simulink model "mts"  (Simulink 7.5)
settings: Solver=FixedStepDiscrete  StartTime=1  StopTime=num(end)  FixedStep=1  RelTol=1e-3
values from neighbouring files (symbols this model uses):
  high = data{2}    [priceTxt.m]
  low = data{3}    [priceTxt.m]
  spread = data{5}    [priceTxt.m]
undefined symbols (not defined in the file or in its folder): sl, tp
libraries: dspsrcs4 x4, dspsigops x1

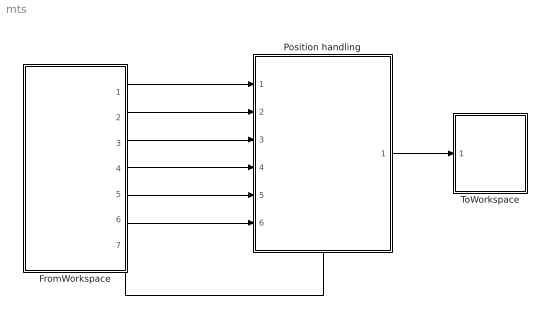
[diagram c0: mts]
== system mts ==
  FromWorkspace : Subsystem
  Position handling : Stateflow chart  TreatAsAtomicUnit=on
  ToWorkspace : Subsystem
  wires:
  FromWorkspace/1(price) -> Position handling/1(Input)
  FromWorkspace/2(spread) -> Position handling/2(spread)
  FromWorkspace/3(high) -> Position handling/3(high)
  FromWorkspace/4(low) -> Position handling/4(low)
  FromWorkspace/5(tp) -> Position handling/5(tp)
  FromWorkspace/6(sl) -> Position handling/6(sl)
  FromWorkspace/7(Buy/Sell) -> Position handling/Trigger
  Position handling/1(Output) -> ToWorkspace/1(In1)

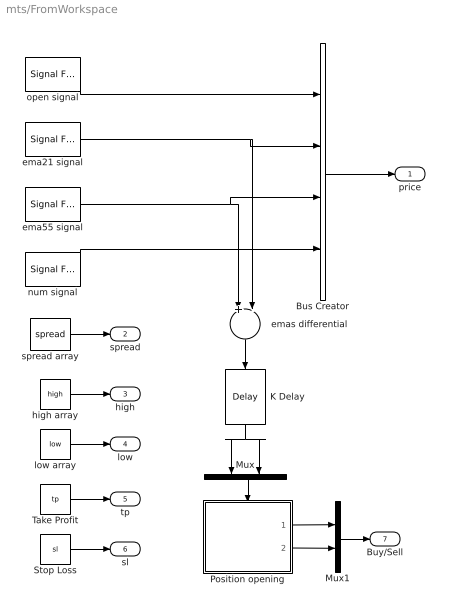
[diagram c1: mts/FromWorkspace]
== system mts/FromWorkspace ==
  Bus Creator : BusCreator  UseBusObject=on
  K Delay : dspsigops/Delay  dly_unit=Samples  delay=K  ic_detail=off  dif_ic_for_ch=off  dif_ic_for_dly=off  ic=0  reset_popup=None
  Mux : Mux  Inputs=2
  Mux1 : Mux  Inputs=2
  Position opening : Stateflow chart  TreatAsAtomicUnit=on
  Stop Loss : Constant  Value=sl  OutDataType=fixdt(1, 16)  OutScaling=2^0
  Take Profit : Constant  Value=tp  OutDataType=fixdt(1, 16)  OutScaling=2^0
  ema21 signal : dspsrcs4/Signal From Workspace  SystemSampleTime=-1  X=ema21  Ts=1  nsamps=1  OutputAfterFinalValue=Holding final value  ignoreOrWarnInputAndFrameLengths=off
  ema55 signal : dspsrcs4/Signal From Workspace  SystemSampleTime=-1  X=ema55  Ts=1  nsamps=1  OutputAfterFinalValue=Holding final value  ignoreOrWarnInputAndFrameLengths=off
  emas differential : Sum  Inputs=+-  OutDataType=fixdt(1, 16)  OutScaling=2^-10
  high array : Constant  Value=high  OutDataType=fixdt(1, 16)  OutScaling=2^0
  low array : Constant  Value=low  OutDataType=fixdt(1, 16)  OutScaling=2^0
  num signal : dspsrcs4/Signal From Workspace  SystemSampleTime=-1  X=num  Ts=1  nsamps=1  OutputAfterFinalValue=Holding final value  ignoreOrWarnInputAndFrameLengths=off
  open signal : dspsrcs4/Signal From Workspace  SystemSampleTime=-1  X=open  Ts=1  nsamps=1  OutputAfterFinalValue=Setting to zero  ignoreOrWarnInputAndFrameLengths=off
  spread array : Constant  Value=spread  OutDataType=fixdt(1, 16)  OutScaling=2^0
  price : Outport  OutDataType=fixdt(1, 16)  OutScaling=2^0
  spread : Outport  Port=2  OutDataType=fixdt(1, 16)  OutScaling=2^0
  high : Outport  Port=3  OutDataType=fixdt(1, 16)  OutScaling=2^0
  low : Outport  Port=4  OutDataType=fixdt(1, 16)  OutScaling=2^0
  tp : Outport  Port=5  OutDataType=fixdt(1, 16)  OutScaling=2^0
  sl : Outport  Port=6  OutDataType=fixdt(1, 16)  OutScaling=2^0
  Buy/Sell : Outport  Port=7  OutDataType=fixdt(1, 16)  OutScaling=2^0
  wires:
  open signal/1 -> Bus Creator/1
  ema21 signal/1 -> Bus Creator/2, emas differential/2
  ema55 signal/1 -> Bus Creator/3, emas differential/1
  num signal/1 -> Bus Creator/4
  spread array/1 -> spread/1
  high array/1 -> high/1
  low array/1 -> low/1
  Take Profit/1 -> tp/1
  Stop Loss/1 -> sl/1
  Bus Creator/1 -> price/1
  emas differential/1 -> K Delay/1
  K Delay/1 -> Mux/2, Mux/1
  Mux/1 -> Position opening/Trigger
  Position opening/1(OpenBuy) -> Mux1/1
  Position opening/2(OpenSell) -> Mux1/2
  Mux1/1 -> Buy/Sell/1

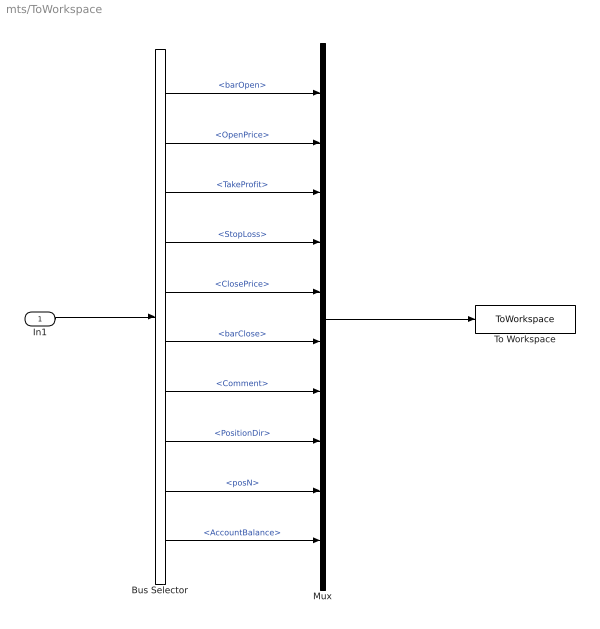
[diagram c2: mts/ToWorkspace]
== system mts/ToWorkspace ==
  In1 : Inport
  Bus Selector : BusSelector  OutputSignals=barOpen,OpenPrice,TakeProfit,StopLoss,ClosePrice,barClose,Comment,PositionDir,posN,AccountBalance
  Mux : Mux  Inputs=10
  To Workspace : ToWorkspace  VariableName=AccountBalance  SampleTime=-1  SaveFormat=Array
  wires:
  In1/1 -> Bus Selector/1
  Mux/1 -> To Workspace/1
  Bus Selector/1 -> Mux/1  "<barOpen>"
  Bus Selector/2 -> Mux/2  "<OpenPrice>"
  Bus Selector/3 -> Mux/3  "<TakeProfit>"
  Bus Selector/4 -> Mux/4  "<StopLoss>"
  Bus Selector/5 -> Mux/5  "<ClosePrice>"
  Bus Selector/6 -> Mux/6  "<barClose>"
  Bus Selector/7 -> Mux/7  "<Comment>"
  Bus Selector/8 -> Mux/8  "<PositionDir>"
  Bus Selector/9 -> Mux/9  "<posN>"
  Bus Selector/10 -> Mux/10  "<AccountBalance>"

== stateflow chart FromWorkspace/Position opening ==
  (default) -> (junction 3)
  (junction 3) -> (junction 4) : Buy{OpenBuy;}
  (junction 3) -> (junction 5) : {OpenSell;}

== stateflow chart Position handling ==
  state Position handling [group]
  (junction 16) -> (junction 17) : {Output.AccountBalance = 100000;}%3
  (default) -> (junction 16) : [Input.num>=56 && Input.num>Output.barClose] {Output.barOpen=Input.num; i = Input.num-1; Output.posN++;}%1
  (junction 16) -> (junction 17) : [Output.posN!=1]%2
  (junction 17) -> (junction 18) : OpenSell {Output.PositionDir=-1; Output.OpenPrice=Input.open; Output.StopLoss=Output.OpenPrice+sl+spread[i]*1e-5; Output.TakeProfit=Output.OpenPrice-tp+spread[i]*1e-5;}%5
  (junction 17) -> (junction 18) : OpenBuy {Output.PositionDir=1; Output.OpenPrice=Input.open+spread[i]*1e-5; Output.StopLoss=Output.OpenPrice-sl-spread[i]*1e-5; Output.TakeProfit=Output.OpenPrice+tp-spread[i]*1e-5;}%4
  (junction 18) -> (junction 20) : [Output.PositionDir==1]%6
  (junction 18) -> (junction 21) : %7
  (junction 20) -> (junction 19) : {Output.ClosePrice = Output.TakeProfit; Output.Comment = 1;} %13
  (junction 21) -> (junction 22) : {Output.ClosePrice = Output.TakeProfit; Output.Comment = 1;} %20
  (junction 20) -> (junction 25) : [low[i] <= Output.StopLoss] {Output.ClosePrice = Output.StopLoss; Output.Comment = -1;} %10
  (junction 28) -> (junction 20) : {i++;}%9
  (junction 19) -> (junction 24) : %14
  (junction 20) -> (junction 28) : [!(high[i] >= Output.TakeProfit)&& !(low[i] <= Output.StopLoss)]%8
  (junction 22) -> (junction 23) : %21
  (junction 21) -> (junction 26) : [(high[i]+spread[i]*1e-5)>= Output.StopLoss] {Output.ClosePrice = Output.StopLoss; Output.Comment = -1;} %17
  (junction 21) -> (junction 27) : [!((low[i]+spread[i]*1e-5) <= Output.TakeProfit) && !((high[i]+spread[i]*1e-5)>= Output.StopLoss)]%15
  (junction 27) -> (junction 21) : {i++;}%16
  (junction 26) -> (junction 23) : %18
  (junction 25) -> (junction 24) : %11
  (junction 23) -> (junction 30) : {posDif = Output.OpenPrice - Output.ClosePrice; Output.AccountBalance = Output.AccountBalance + Lots*100000*posDif; Output.barClose=i+1;}%19
  (junction 24) -> (junction 29) : {posDif = Output.ClosePrice - Output.OpenPrice; Output.AccountBalance = Output.AccountBalance + Lots*100000*posDif; Output.barClose=i+1;}%12
